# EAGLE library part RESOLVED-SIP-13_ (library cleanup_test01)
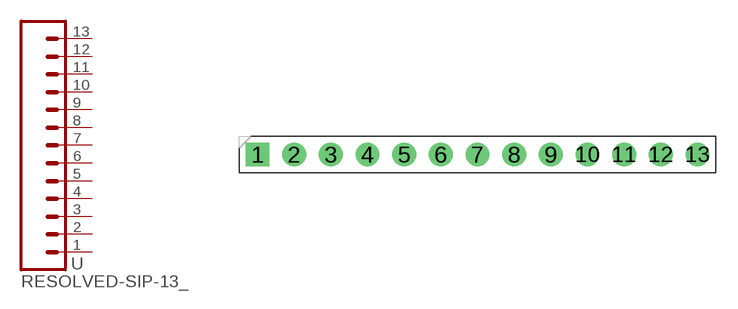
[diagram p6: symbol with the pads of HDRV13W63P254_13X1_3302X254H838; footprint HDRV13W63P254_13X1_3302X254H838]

Designator prefix -

## RESOLVED-SIP-13_2.54-SPACE-VERTICAL  [HDRV13W63P254_13X1_3302X254H838]
1  1  pas
2  2  pas
3  3  pas
4  4  pas
5  5  pas
6  6  pas
7  7  pas
8  8  pas
9  9  pas
10  10  pas
11  11  pas
12  12  pas
13  13  pas

## Footprint HDRV13W63P254_13X1_3302X254H838 (pad centres in mm)
drill 1.1 pad 1.65 square: 1 0,0
drill 1.1 pad 1.65: 2 2.54,0; 3 5.08,0; 4 7.62,0; 5 10.16,0; 6 12.7,0; 7 15.24,0; 8 17.78,0; 9 20.32,0; 10 22.86,0; 11 25.4,0; 12 27.94,0; 13 30.48,0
